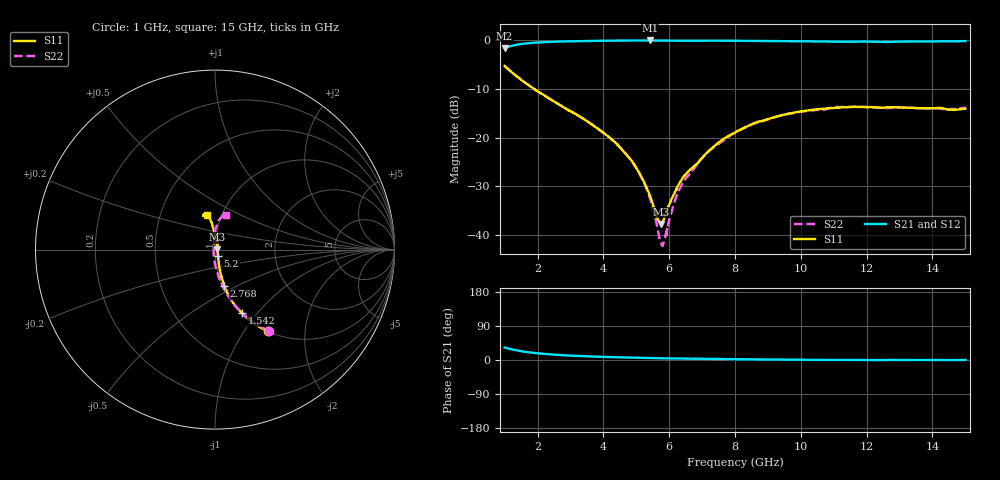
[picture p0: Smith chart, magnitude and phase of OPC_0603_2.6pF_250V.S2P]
! FILE NAME
! DATE 08/14/2012  14:53
! CORRECTED  DATA
# GHz  S  MA  R  50.00
!  FREQ  S11M  S11A  S21M  S21A  S12M  S12A  S22M  S22A
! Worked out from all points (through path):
!   1601 points, 1 GHz to 15 GHz, reference 50 ohm
!   highest |S21| = -0.04 dB at 5.419 GHz (marker M1); lowest = -1.6 dB at 1 GHz (marker M2)
!   group delay of S21, straight-line fit = 3.93 ps
!   lowest |S11| = -37.8 dB at 5.76 GHz (marker M3), VSWR 1.03, Z = 51.3 + j0.104 ohm
!   |S11| at or under -10 dB: 1.895 GHz to end of sweep
!   |S22| runs from -42.4 to -5.3 dB; largest |S21 - S12| = 0.01
!   S11 on the Smith chart (normalised r, x): 1 GHz: 1.00, -1.30; 1.542 GHz: 1.00, -0.83; 2.768 GHz: 1.02, -0.43; 5.2 GHz: 1.03, -0.07; 15 GHz: 0.85, +0.34
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1  0.5442 -56.9  0.8341 33.1  0.8333 33.0  0.5445 -56.4
1.5425  0.3833 -67.1  0.919 22.7  0.9174 22.6  0.3835 -66.8
2.05  0.2921 -72.3  0.9521 17.3  0.9513 17.2  0.2921 -72.6
2.7675  0.2081 -75.7  0.9735 12.7  0.9722 12.6  0.2076 -78.1
3.33625  0.1603 -76.7  0.9827 10.3  0.9811 10.2  0.1599 -81.5
4.49125  0.08016 -74.6  0.9929 7.0  0.9919 6.9  0.08016 -90.1
4.885  0.05614 -71.0  0.9942 6.2  0.9931 6.1  0.05556 -94.4
5.2  0.03697 -63.8  0.9948 5.6  0.9936 5.4  0.03605 -100.1
5.41875  0.02494 -54.0  0.9959 5.1  0.9939 5.0  0.02352 -108.9
5.55875  0.01812 -38.8  0.9948 4.9  0.994 4.8  0.01583 -120.2
5.6725  0.01401 -18.1  0.9948 4.7  0.9939 4.6  0.01028 -141.6
5.76  0.01288 4.5  0.9946 4.5  0.9933 4.4  0.0081 -172.7
5.8475  0.01475 27.2  0.9937 4.4  0.9923 4.3  0.008725 146.8
6.18  0.02777 61.4  0.9909 4.0  0.9896 3.9  0.02274 101.8
6.4425  0.03986 69.8  0.9887 3.7  0.9874 3.6  0.03521 93.0
7.1425  0.06975 87.9  0.9906 3.2  0.9894 3.1  0.06956 92.0
8  0.1127 94.2  0.989 2.2  0.9876 2.1  0.1113 88.6
9.155  0.1604 98.1  0.9813 1.2  0.9798 1.1  0.1592 83.0
10.33625  0.1923 101.3  0.9745 0.4  0.9732 0.3  0.1898 77.7
11.05375  0.202 103.4  0.9673 0.3  0.966 0.1  0.2053 75.8
12.6725  0.204 108.3  0.9606 0.1  0.9593 -0.0  0.2009 72.0
15  0.1983 102.9  0.9802 0.2  0.9789 0.1  0.2035 72.2
